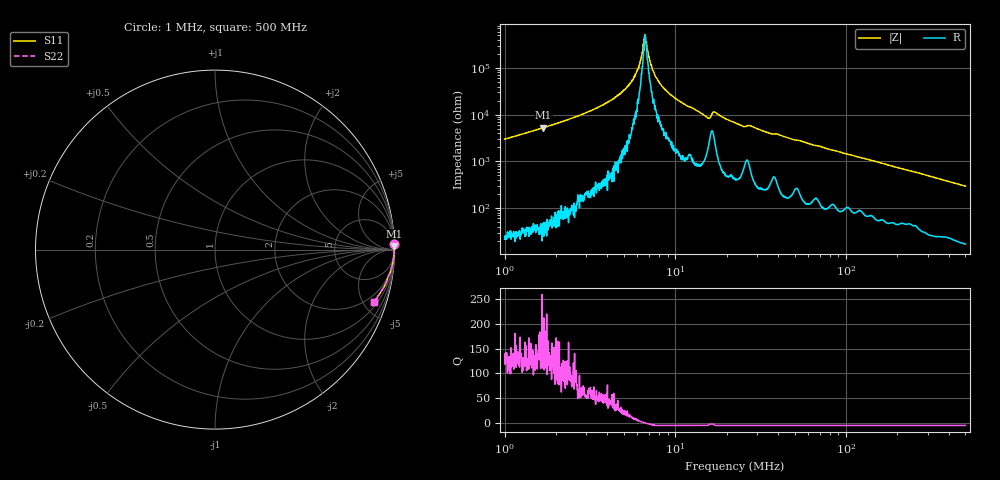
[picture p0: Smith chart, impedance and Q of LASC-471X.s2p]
!s-Parameter Generated by FASTRON Sdn. Bhd.
!FASTRON P/N : LASC-471X
!Keysight Technologies,E4991B,MY54100416,A.01.15
!Date: Tue Mar 17 16:07:17 2026
!Version  : Rev00 Tue Mar 17 16:07:17 2026
!Data & Calibration Information:
!PortZ  Port1:50+j0  Port2:50+j0
!When reading, reference impedance value at option line is always used.
! Remarks : This data is being provided solely for informational purposes.
!Freq	S11	S21	S12	S22
# Hz S dB R 50
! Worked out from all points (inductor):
!   1601 points, 1 MHz to 500 MHz, reference 50 ohm
!   read as one part in series: L = 464 uH near 1.032 MHz
!   highest Q = 166 at 1.683 MHz (marker M1), where L = 497 uH
!   self-resonance near 6.656 MHz
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1000000  -0.01 1.9  -29.51 -87.7  -29.51 -87.7  -0.01 1.9
1682824  -0.00 1.1  -34.42 -88.4  -34.42 -88.4  -0.00 1.1
2820919  -0.00 0.6  -40.07 -88.6  -40.07 -88.6  -0.00 0.6
4127647  -0.00 0.3  -45.84 -88.3  -45.84 -88.3  -0.00 0.3
5210914  -0.00 0.1  -51.80 -85.9  -51.80 -85.9  -0.00 0.1
5631849  -0.00 0.1  -54.78 -83.6  -54.78 -83.6  -0.00 0.1
5969719  -0.00 0.1  -58.85 -82.2  -58.85 -82.2  -0.00 0.1
6230305  -0.00 0.0  -63.04 -73.6  -63.04 -73.6  -0.00 0.0
6477059  -0.00 0.0  -69.84 -55.6  -69.84 -55.6  -0.00 0.0
6655579  -0.00 0.0  -72.30 -9.5  -72.30 -9.5  -0.00 0.0
6786098  -0.00 -0.0  -71.19 41.7  -71.19 41.7  -0.00 -0.0
7054865  -0.00 -0.0  -64.01 68.0  -64.01 68.0  -0.00 -0.0
7334276  -0.00 -0.1  -59.59 75.5  -59.59 75.5  -0.00 -0.1
7957584  -0.00 -0.1  -54.41 81.2  -54.41 81.2  -0.00 -0.1
9852770  -0.00 -0.2  -47.35 85.2  -47.35 85.2  -0.00 -0.2
1.534122e7  -0.02 -0.6  -38.85 79.2  -38.85 79.2  -0.02 -0.6
1.58254e7  -0.03 -0.6  -38.43 70.6  -38.43 70.6  -0.03 -0.6
1.703747e7  -0.02 -0.5  -41.12 76.7  -41.12 76.7  -0.02 -0.5
2.236068e7  -0.01 -0.9  -36.55 85.6  -36.55 85.6  -0.01 -0.9
6.307767e7  -0.03 -2.5  -27.18 84.1  -27.18 84.1  -0.03 -2.5
1.77937e8  -0.12 -6.8  -18.47 79.9  -18.47 79.9  -0.12 -6.8
5e8  -0.62 -18.4  -10.01 68.3  -10.01 68.3  -0.62 -18.4
